(* Logix 5000 Routine export TimeSync; software revision 19.01 *)

TYPE AparianTimeSyncDateTime :
STRUCT
   UTC : LINT;
   Year : INT;
   Month : SINT;
   Day : SINT;
   Hour : SINT;
   Minute : SINT;
   Second : SINT;
   Nanosecond : DINT;
END_STRUCT
END_TYPE

TYPE AparianTimeSyncVelocity :
STRUCT
   TrueCourseOverGround : REAL;
   SpeedOverGroundKnots : REAL;
   SpeedOverGroundKmh : REAL;
END_STRUCT
END_TYPE

TYPE AparianTimeSyncStatusR02 :
STRUCT
   ConfigurationValid : BOOL;
   PTPEnabled : BOOL;
   NTPEnabled : BOOL;
   AntennaShort : BOOL;
   Fix2D : BOOL;
   Fix3D : BOOL;
   FixAutonomous : BOOL;
   FixDifferential : BOOL;
   NTPSource1Connected : BOOL;
   NTPSource2Connected : BOOL;
END_STRUCT
END_TYPE

TYPE AparianTimeSyncOutput :
STRUCT
   ReferenceLatitude : REAL;
   ReferenceLongtitude : REAL;
   ReferenceAltitude : REAL;
END_STRUCT
END_TYPE

TYPE AparianTimeSyncAccuracy :
STRUCT
   PDOP : REAL;
   HDOP : REAL;
   VDOP : REAL;
   LatitudeError : REAL;
   LongtitudeError : REAL;
   AltitudeError : REAL;
END_STRUCT
END_TYPE

TYPE AparianTimeSyncPosition :
STRUCT
   Latitude : REAL;
   Longtitude : REAL;
   Altitude : REAL;
   ReferenceLatitude : REAL;
   ReferenceLongtitude : REAL;
   ReferenceAltitude : REAL;
   RelativeLatitude : REAL;
   RelativeLongtitude : REAL;
   RelativeAltitude : REAL;
   RelativeNorth : REAL;
   RelativeEast : REAL;
END_STRUCT
END_TYPE

TYPE AparianTimeSyncInput :
STRUCT
   Instance : STRING;
   Status : AparianTimeSyncStatusR02;
   InterferenceIndication : REAL;
   SatelliteCount : SINT;
   DateTime : AparianTimeSyncDateTime;
   Velocity : AparianTimeSyncVelocity;
   Position : AparianTimeSyncPosition;
   Odometer : AparianTimeSyncOdometer;
   Accuracy : AparianTimeSyncAccuracy;
END_STRUCT
END_TYPE

TYPE AparianTimeSyncOdometer :
STRUCT
   DistanceSinceReset : DINT;
   DistanceTotal : DINT;
   DistanceAccuracy : DINT;
END_STRUCT
END_TYPE

VAR_GLOBAL   (* controller tags *)
   TSM01Output : AparianTimeSyncOutput;
   TimeSyncResetOdometer : BOOL;
   TSM01Input : AparianTimeSyncInput;
   ResetOdometer : MESSAGE;
        MessageParameters(MessageType := CIP Generic, ConnectedFlag := 2, ConnectionPath := TSM01, ServiceCode := 16#0076, ObjectType := 16#040a, TargetObject := 1)
END_VAR

PROGRAM MainProgram

ROUTINE TimeSync   (* ladder *)
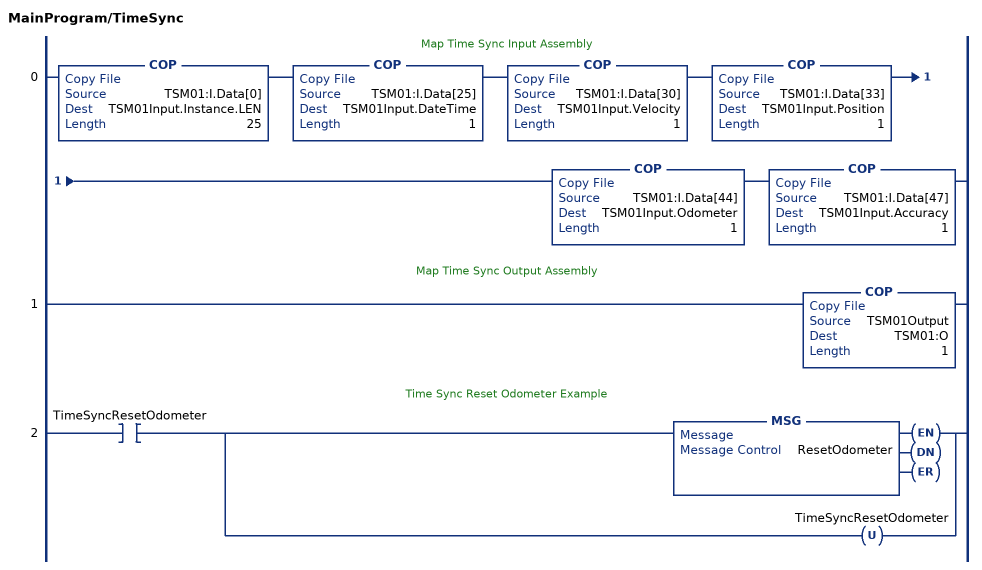
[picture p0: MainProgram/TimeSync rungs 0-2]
   // Map Time Sync Input Assembly
   0: COP(TSM01:I.Data[0],TSM01Input.Instance.LEN,25)COP(TSM01:I.Data[25],TSM01Input.DateTime,1)COP(TSM01:I.Data[30],TSM01Input.Velocity,1)COP(TSM01:I.Data[33],TSM01Input.Position,1)COP(TSM01:I.Data[44],TSM01Input.Odometer,1)COP(TSM01:I.Data[47],TSM01Input.Accuracy,1);
   // Map Time Sync Output Assembly
   1: COP(TSM01Output,TSM01:O,1);
   // Time Sync Reset Odometer Example
   2: XIC(TimeSyncResetOdometer)[MSG(ResetOdometer) ,OTU(TimeSyncResetOdometer) ];
END_ROUTINE
END_PROGRAM
